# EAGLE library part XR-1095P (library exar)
EQUALIZER DISPLAY/FILTER/MULTIPLEXER
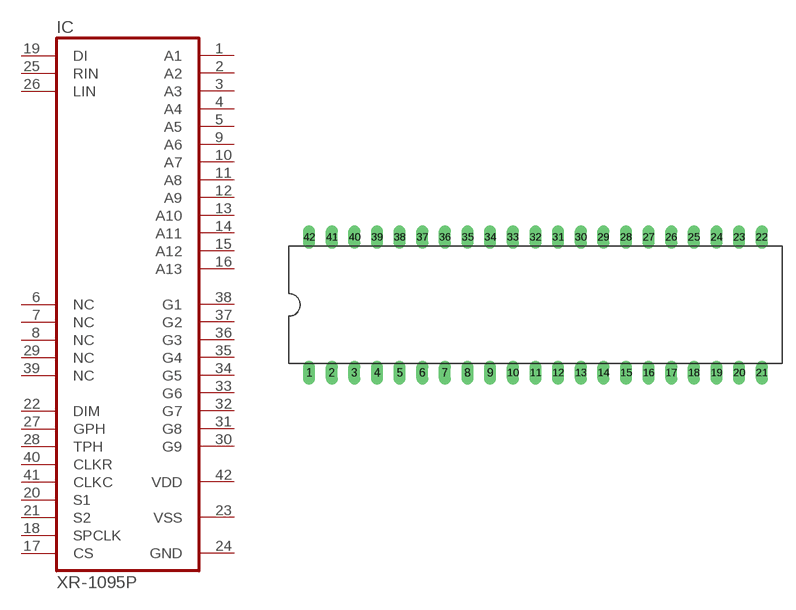
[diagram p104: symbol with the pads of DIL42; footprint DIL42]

Designator prefix IC

## XR-1095P (OC_FARNELL: unknown; OC_NEWARK: unknown)  [DIL42]
1  A1  out
2  A2  out
3  A3  out
4  A4  out
5  A5  out
6  NC  nc
7  NC  nc
8  NC  nc
9  A6  out
10  A7  out
11  A8  out
12  A9  out
13  A10  out
14  A11  out
15  A12  out
16  A13  out
17  CS  in
18  SPCLK  in
19  DI  in
20  S1  in
21  S2  in
22  DIM  in
23  VSS  pwr
24  GND  pwr
25  RIN  in
26  LIN  in
27  GPH  in
28  TPH  in
29  NC  nc
30  G9  out
31  G8  out
32  G7  out
33  G6  out
34  G5  out
35  G4  out
36  G3  out
37  G2  out
38  G1  out
39  NC  nc
40  CLKR  in
41  CLKC  in
42  VDD  pwr

## Footprint DIL42 (pad centres in mm)
Dual In Line Package
drill 0.813 long: 1 -25.4,-7.62; 2 -22.86,-7.62; 3 -20.32,-7.62; 4 -17.78,-7.62; 5 -15.24,-7.62; 6 -12.7,-7.62; 7 -10.16,-7.62; 8 -7.62,-7.62; 9 -5.08,-7.62; 10 -2.54,-7.62; 11 0,-7.62; 12 2.54,-7.62; 13 5.08,-7.62; 14 7.62,-7.62; 15 10.16,-7.62; 16 12.7,-7.62; 17 15.24,-7.62; 18 17.78,-7.62; 19 20.32,-7.62; 20 22.86,-7.62; 21 25.4,-7.62; 22 25.4,7.62; 23 22.86,7.62; 24 20.32,7.62; 25 17.78,7.62; 26 15.24,7.62; 27 12.7,7.62; 28 10.16,7.62; 29 7.62,7.62; 30 5.08,7.62; 31 2.54,7.62; 32 0,7.62; 33 -2.54,7.62; 34 -5.08,7.62; 35 -7.62,7.62; 36 -10.16,7.62; 37 -12.7,7.62; 38 -15.24,7.62; 39 -17.78,7.62; 40 -20.32,7.62; 41 -22.86,7.62; 42 -25.4,7.62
